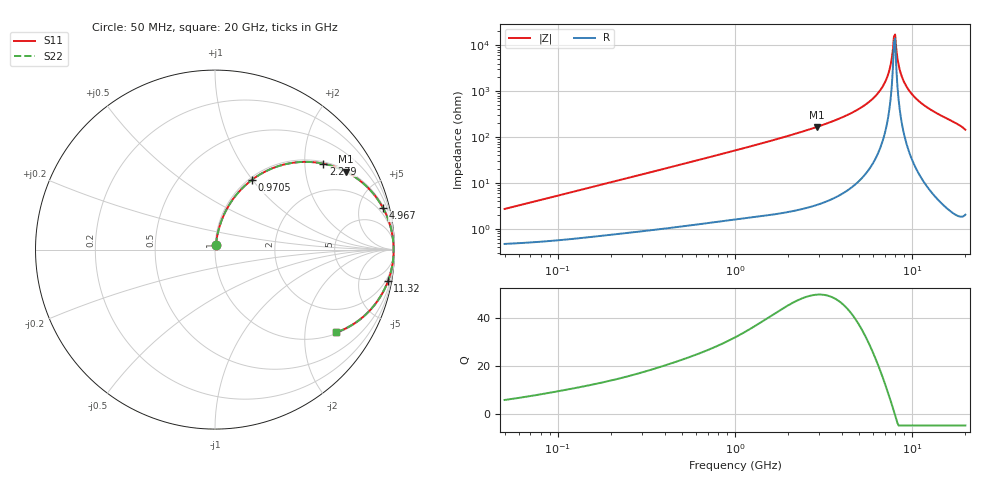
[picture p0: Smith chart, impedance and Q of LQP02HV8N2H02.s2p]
!Murata Part Number: LQP02HV8N2H02
!These Parameters are Measured in Series Mode Connection
!  o--[Z]--o
!Port1  Port2
!  o-------o
!Freq. Start=50[MHz] Stop=20[GHz], 401[Steps]
# Hz S RI R 50
!Freq.(Hz) S11(Real) S11(Imag) S21(Real) S21(Imag) S12(Real) S12(Imag) S22(Real) S22(Imag)
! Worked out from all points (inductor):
!   401 points, 50 MHz to 20 GHz, reference 50 ohm
!   read as one part in series: L = 8.53 nH near 51.52 MHz
!   highest Q = 49.9 at 2.896 GHz (marker M1), where L = 9.15 nH
!   self-resonance near 7.902 GHz
!   S11 on the Smith chart (normalised r, x): 50 MHz: 1.01, +0.05; 970.5 MHz: 1.03, +0.99; 2.279 GHz: 1.05, +2.48; 4.967 GHz: 1.21, +8.08; 11.32 GHz: 1, -11; 20 GHz: 1.04, -2.89
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5e7  0.00544 0.0267  0.9946 -0.0267  0.9946 -0.0267  0.00544 0.0267
1.364002e8  0.0114 0.0706  0.9886 -0.0706  0.9886 -0.0706  0.0114 0.0706
3.721004e8  0.0441 0.1812  0.9559 -0.1812  0.9559 -0.1812  0.0441 0.1812
9.70487e8  0.2056 0.3885  0.7944 -0.3885  0.7944 -0.3885  0.2056 0.3885
1e9  0.2152 0.3956  0.7848 -0.3956  0.7848 -0.3956  0.2152 0.3956
2.279204e9  0.6042 0.4786  0.3958 -0.4786  0.3958 -0.4786  0.6042 0.4786
2.728004e9  0.7006 0.448  0.2994 -0.448  0.2994 -0.448  0.7006 0.448
2.896447e9  0.7311 0.4335  0.2689 -0.4335  0.2689 -0.4335  0.7311 0.4335
4.966507e9  0.9369 0.2304  0.0631 -0.2304  0.0631 -0.2304  0.9369 0.2304
5.769027e9  0.9679 0.1598  0.0321 -0.1598  0.0321 -0.1598  0.9679 0.1598
6.503449e9  0.9843 0.1013  0.0157 -0.1013  0.0157 -0.1013  0.9843 0.1013
7.009217e9  0.9908 0.0642  0.00925 -0.0642  0.00925 -0.0642  0.9908 0.0642
7.442007e9  0.9939 0.0343  0.00611 -0.0343  0.00611 -0.0343  0.9939 0.0343
7.784049e9  0.995 0.0118  0.00496 -0.0118  0.00496 -0.0118  0.995 0.0118
8.020766e9  0.9952 -0.0033  0.00476 0.0033  0.00476 0.0033  0.9952 -0.0033
8.141811e9  0.9952 -0.0108  0.00484 0.0108  0.00484 0.0108  0.9952 -0.0108
8.516016e9  0.9942 -0.0335  0.00576 0.0335  0.00576 0.0335  0.9942 -0.0335
9.041845e9  0.9914 -0.0637  0.00863 0.0637  0.00863 0.0637  0.9914 -0.0637
9.892087e9  0.9835 -0.1091  0.0165 0.1091  0.0165 0.1091  0.9835 -0.1091
1.131968e10  0.9633 -0.1769  0.0367 0.1769  0.0367 0.1769  0.9633 -0.1769
1.621653e10  0.8486 -0.3531  0.1514 0.3531  0.1514 0.3531  0.8486 -0.3531
2e10  0.6742 -0.4616  0.3258 0.4616  0.3258 0.4616  0.6742 -0.4616
